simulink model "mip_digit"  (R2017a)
settings: Solver=VariableStepAuto  StartTime=0.0  StopTime=50.0  RelTol=1e-3
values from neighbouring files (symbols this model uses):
  g = 9.81    [analisi_linearizzato.m]
  Ir = 10    [analisi_linearizzato.m]
  Iw = 0.06    [analisi_linearizzato.m]
  L = 0.4    [analisi_linearizzato.m]
  mr = 3    [analisi_linearizzato.m]
  mw = 20    [analisi_linearizzato.m]
  R = 0.2    [analisi_linearizzato.m]
  R1d = c2d(R1,Ts,'tustin')    [analisi_linearizzato.m]
  R2d = c2d(R2,Ts,'tustin')    [analisi_linearizzato.m]
  Ts = 2*pi/(50*0.5)    (= 0.251327412287)    [analisi_linearizzato.m]
undefined symbols (not defined in the file or in its folder): magnitude

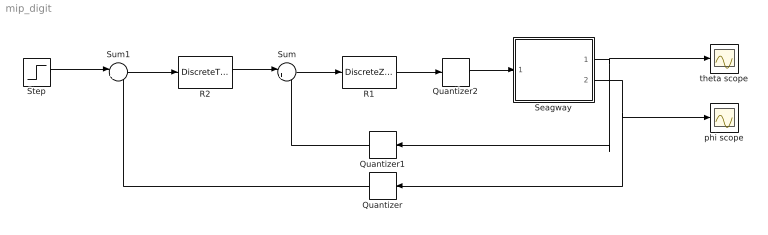
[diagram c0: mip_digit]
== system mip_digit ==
  Quantizer : Quantizer  QuantizationInterval=2*pi/2^12
  Quantizer1 : Quantizer  QuantizationInterval=2*pi/2^12
  Quantizer2 : Quantizer  QuantizationInterval=10/2^14
  R1 : DiscreteZeroPole  Zeros=R1d.z{1}  Poles=R1d.p{1}  Gain=R1d.k  SampleTime=Ts
  R2 : DiscreteTransferFcn  Numerator=R2d.num{1}  Denominator=R2d.den{1}  SampleTime=Ts
  Seagway : Subsystem
  Step : Step  Time=2  After=10*pi/180  SampleTime=0
  Sum : Sum  Inputs=|+-
  Sum1 : Sum  Inputs=|+-
  phi scope : Scope
  theta scope : Scope
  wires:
  Sum/1 -> R1/1
  R1/1 -> Quantizer2/1
  Seagway/1(Theta) -> Quantizer1/1, theta scope/1
  Sum1/1 -> R2/1
  Seagway/2(Phi) -> Quantizer/1, phi scope/1
  Step/1 -> Sum1/1
  R2/1 -> Sum/1
  Quantizer/1 -> Sum1/2
  Quantizer1/1 -> Sum/2
  Quantizer2/1 -> Seagway/1(Tau)

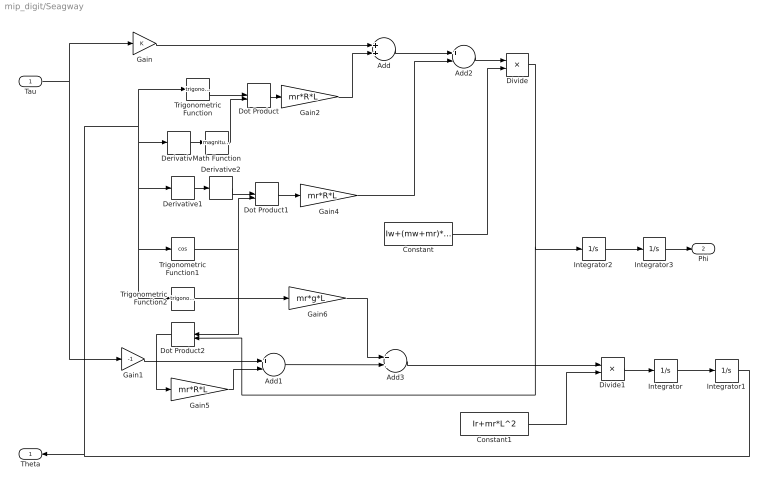
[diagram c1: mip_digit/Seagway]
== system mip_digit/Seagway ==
  Tau : Inport
  Add : Sum
  Add1 : Sum  Inputs=+-
  Add2 : Sum  Inputs=+-
  Add3 : Sum
  Constant : Constant  Value=Iw+(mw+mr)*R^2
  Constant1 : Constant  Value=Ir+mr*L^2
  Derivative : Derivative
  Derivative1 : Derivative
  Derivative2 : Derivative
  Divide : Product  Inputs=*/
  Divide1 : Product  Inputs=*/
  Dot Product : DotProduct
  Dot Product1 : DotProduct
  Dot Product2 : DotProduct
  Gain : Gain
  Gain1 : Gain  Gain=-1
  Gain2 : Gain  Gain=mr*R*L
  Gain4 : Gain  Gain=mr*R*L
  Gain5 : Gain  Gain=mr*R*L
  Gain6 : Gain  Gain=mr*g*L
  Integrator{,1..3} (4 alike) : Integrator
  Math Function : Math  Operator=magnitude^2
  Trigonometric Function : Trigonometry
  Trigonometric Function1 : Trigonometry  Operator=cos
  Trigonometric Function2 : Trigonometry
  Theta : Outport
  Phi : Outport  Port=2
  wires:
  Add1/1 -> Add3/2
  Integrator3/1 -> Phi/1
  Integrator2/1 -> Integrator3/1
  Divide1/1 -> Integrator/1
  Integrator/1 -> Integrator1/1
  Derivative2/1 -> Dot Product1/1
  Add/1 -> Add2/1
  Divide/1 -> Dot Product2/2, Integrator2/1
  Derivative/1 -> Math Function/1
  Dot Product1/1 -> Gain4/1
  Trigonometric Function1/1 -> Dot Product1/2, Dot Product2/1
  Derivative1/1 -> Derivative2/1
  Integrator1/1 -> Trigonometric Function1/1, Trigonometric Function2/1, Derivative1/1, Derivative/1, Trigonometric Function/1, Theta/1
  Math Function/1 -> Dot Product/2
  Add2/1 -> Divide/1
  Gain5/1 -> Add1/2
  Constant/1 -> Divide/2
  Gain1/1 -> Add1/1
  Add3/1 -> Divide1/1
  Dot Product2/1 -> Gain5/1
  Trigonometric Function/1 -> Dot Product/1
  Tau/1 -> Gain/1, Gain1/1
  Gain4/1 -> Add2/2
  Trigonometric Function2/1 -> Gain6/1
  Dot Product/1 -> Gain2/1
  Gain6/1 -> Add3/1
  Gain2/1 -> Add/2
  Gain/1 -> Add/1
  Constant1/1 -> Divide1/2
